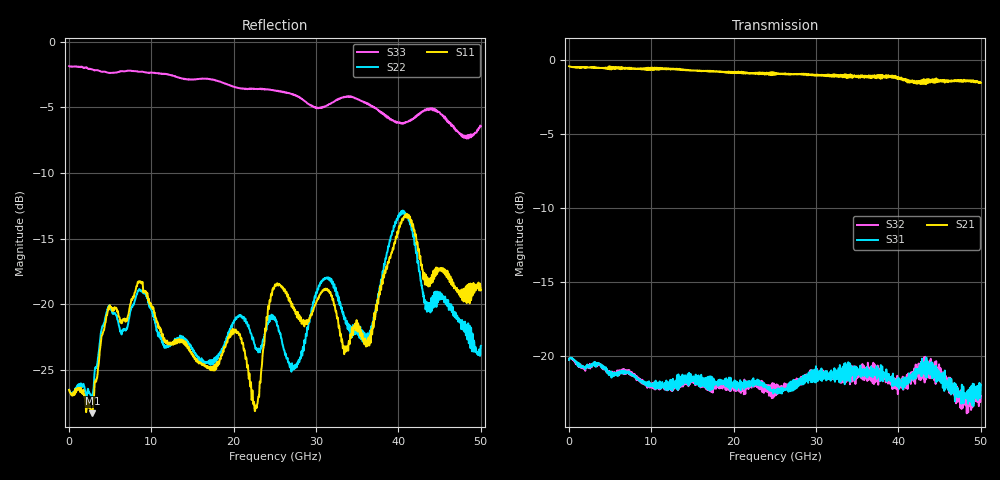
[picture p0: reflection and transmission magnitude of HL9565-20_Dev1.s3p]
! 10/7/2020 1:05:54 PM
! H:\PRODUCTION_DATA\TEMP_S3P.S3P
! CHANNEL.1
! TR.MEASUREMENT
! CORRECTED.DATA
# GHZ S RI R 50.0
! FREQ.GHZ  S11RE  S11IM  S12RE  S12IM  S13RE  S13IM
!  S21RE  S21IM  S22RE  S22IM  S23RE  S23IM
!  S31RE  S31IM  S32RE  S32IM  S33RE  S33IM
!; PortSelection: Port_123
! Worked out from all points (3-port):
!   1429 points, 35 MHz to 50.02 GHz, reference 50 ohm
!   strongest paths, dB at 35 MHz, 12.53 GHz, 25.02 GHz, 37.52 GHz, 50.02 GHz:
!     S21: -0.5, -0.7, -0.9, -1.2, -1.6
!     S31: -20.2, -22.0, -22.3, -20.8, -21.9
!     S32: -20.3, -22.1, -22.3, -21.4, -22.7
!   lowest |S11| = -28.3 dB at 2.87 GHz (marker M1), VSWR 1.08, Z = 49.4 + j3.79 ohm
!   |S11| at or under -10 dB: start of sweep to end of sweep
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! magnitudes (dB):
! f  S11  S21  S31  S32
! 35 MHz  -26.5  -0.5  -20.2  -20.3
! 2.87 GHz  -28.3  -0.5  -20.5  -20.5
! 4.795 GHz  -20.3  -0.5  -21.1  -21.0
! 8.61 GHz  -18.3  -0.6  -21.6  -21.5
! 20.51 GHz  -22.1  -0.9  -21.9  -22.3
! 22.68 GHz  -27.7  -1.0  -21.7  -21.8
! 25.02 GHz  -18.6  -0.9  -22.3  -22.3
! 36.26 GHz  -23.2  -1.1  -21.4  -21.4
! 40.56 GHz  -13.6  -1.3  -22.2  -22.1
! 50.02 GHz  -18.9  -1.6  -21.9  -22.7
